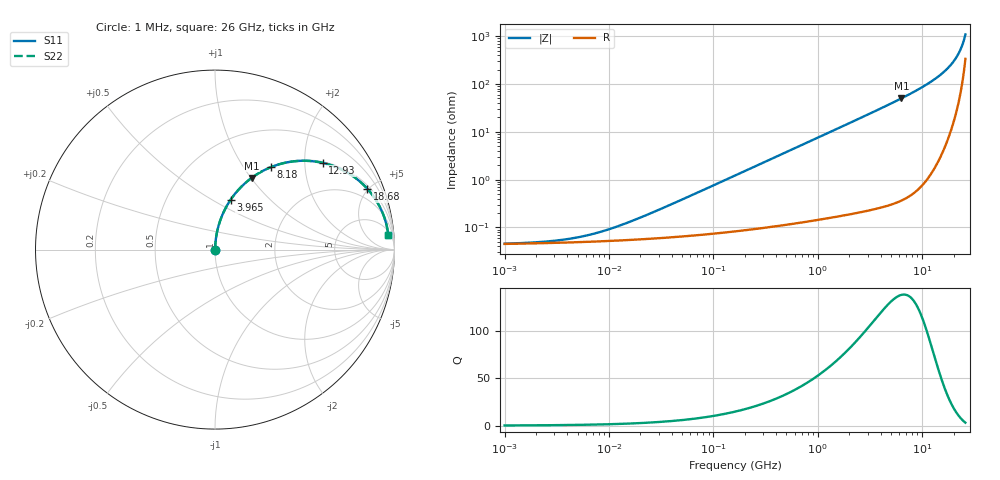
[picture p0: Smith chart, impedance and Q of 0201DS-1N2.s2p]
# MHz S MA R 50
!Freq  MagS11  AngS11  MagS21  AngS21  MagS12  AngS12  MagS22  AngS22
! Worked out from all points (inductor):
!   801 points, 1 MHz to 26 GHz, reference 50 ohm
!   read as one part in series: L = 1.2 nH near 23.07 MHz
!   highest Q = 138 at 6.344 GHz (marker M1), where L = 1.26 nH
!   S11 on the Smith chart (normalised r, x): 1 MHz: 1.00, +0.00; 3.965 GHz: 1.01, +0.61; 8.18 GHz: 1.01, +1.34; 12.93 GHz: 1.03, +2.45; 18.68 GHz: 1.20, +4.93; 26 GHz: 8, +21
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1  0.000458 9.5  0.9995 -0.0  0.9995 -0.0  0.000458 9.5
2.660365  0.0005128 23.0  0.9995 -0.0  0.9995 -0.0  0.0005128 23.0
5.489187  0.0006449 39.9  0.9995 -0.0  0.9995 -0.0  0.0006449 39.9
7.834876  0.0007798 49.2  0.9995 -0.0  0.9995 -0.0  0.0007798 49.2
11.4708  0.001013 58.5  0.9995 -0.0  0.9995 -0.0  0.001013 58.5
29.75071  0.002319 75.0  0.9994 -0.1  0.9994 -0.1  0.002319 75.0
161.2452  0.01218 85.4  0.9991 -0.7  0.9991 -0.7  0.01218 85.4
885.1048  0.06657 85.0  0.9964 -3.8  0.9964 -3.8  0.06657 85.0
1970.942  0.1474 80.8  0.9872 -8.5  0.9872 -8.5  0.1474 80.8
3964.636  0.2909 72.6  0.9543 -16.9  0.9543 -16.9  0.2909 72.6
4797.158  0.348 69.2  0.9348 -20.4  0.9348 -20.4  0.348 69.2
6344.477  0.4483 63.0  0.8906 -26.6  0.8906 -26.6  0.4483 63.0
8180.317  0.5559 55.8  0.8271 -33.8  0.8271 -33.8  0.5559 55.8
10547.38  0.6745 47.1  0.732 -42.4  0.732 -42.4  0.6745 47.1
12925.4  0.7701 38.9  0.6278 -50.4  0.6278 -50.4  0.7701 38.9
15839.57  0.8571 29.7  0.4963 -59.0  0.4963 -59.0  0.8571 29.7
18684.73  0.9141 21.7  0.3707 -66.0  0.3707 -66.0  0.9141 21.7
20684.09  0.9403 16.6  0.2866 -69.8  0.2866 -69.8  0.9403 16.6
22322.8  0.9548 12.7  0.2211 -71.9  0.2211 -71.9  0.9548 12.7
23486.79  0.9618 10.1  0.1768 -72.5  0.1768 -72.5  0.9618 10.1
25027.48  0.9674 6.8  0.1213 -71.0  0.1213 -71.0  0.9674 6.8
26000  0.969 4.8  0.08873 -67.2  0.08873 -67.2  0.969 4.8
